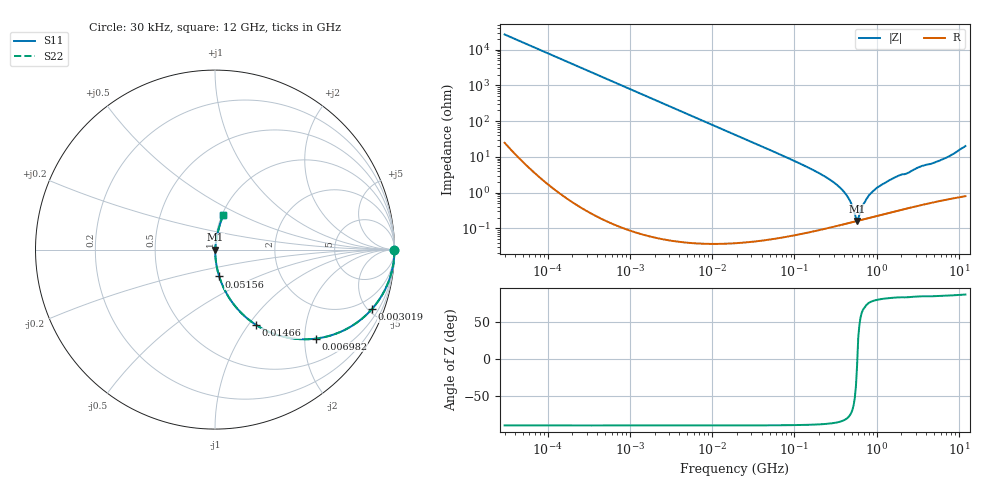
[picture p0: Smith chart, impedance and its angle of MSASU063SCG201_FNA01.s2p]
! MSASU063SCG201_FNA01  S-PARAMETER MODEL  ( General Type )
! Model Generated by TAIYO YUDEN Corporation (http://www.ty-top.com)
! Version 1.0
! TAIYO YUDEN Control No. 140905
! Copyright(c) 2014 TAIYO YUDEN CO.,LTD. All Rights Reserved.
! Product Description (link to TY-COMPAS)
! https://ds.yuden.co.jp/TYCOMPAS/or/detail?pn=MSASU063SCG201JFNA01&u=M
! Products Name : Multilayer Ceramic Capacitors
! Characteristics :
!  Capacitance : 200 pF , Rated Voltage : 50V , TCC : CG / C0G
!  Case Size : 0.6 x 0.3 / 0.024 x 0.012 [mm/inch] , Thickness : 0.3 / 0.012 [mm/inch]
!  (Conditions: Temperature = 25 degC , DC Bias Current/Voltage = 0A / 0V)
! External Node Assignments :
!  1  o---| |---o  2
! GND o---------o GND
! Frequency Range : 0.03MHz  -  12000MHz  [ 401 STEP ]
# MHz S RI R 50
! Freq[MHz].  S11 Real  S11 Imag  S21 Real  S21 Imag  S12 Real  S12 Imag  S22 Real  S22 Imag
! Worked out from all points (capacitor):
!   401 points, 30 kHz to 12 GHz, reference 50 ohm
!   read as one part in series: C = 200 pF near 32 kHz
!   lowest |Z| = 163 mohm at 579 MHz (marker M1)
!   series resonance near 582.7 MHz, so ESL is about 370 pH
!   S11 on the Smith chart (normalised r, x): 30 kHz: open; 3.019 MHz: 1.00, -5.26; 6.982 MHz: 1.00, -2.28; 14.66 MHz: 1.00, -1.08; 51.56 MHz: 1.00, -0.31; 12 GHz: 1.02, +0.40
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0.03  1 -0.00378  1.78e-05 0.00378  1.78e-05 0.00378  1 -0.00378
0.260295  0.9989 -0.0327  0.00108 0.0327  0.00108 0.0327  0.9989 -0.0327
0.886466  0.9877 -0.1102  0.0123 0.1102  0.0123 0.1102  0.9877 -0.1102
2.258455  0.9252 -0.263  0.0748 0.263  0.0748 0.263  0.9252 -0.263
3.018962  0.8738 -0.332  0.1262 0.332  0.1262 0.332  0.8738 -0.332
6.982189  0.5641 -0.4957  0.4359 0.4957  0.4359 0.4957  0.5641 -0.4957
14.65919  0.227 -0.4185  0.773 0.4185  0.773 0.4185  0.227 -0.4185
18.97367  0.1491 -0.3558  0.8509 0.3558  0.8509 0.3558  0.1491 -0.3558
51.55976  0.0233 -0.1493  0.9767 0.1493  0.9767 0.1493  0.0233 -0.1493
164.6252  0.00278 -0.0443  0.9972 0.0443  0.9972 0.0443  0.00278 -0.0443
275.7901  0.00156 -0.0223  0.9984 0.0223  0.9984 0.0223  0.00156 -0.0223
380.7415  0.00142 -0.012  0.9986 0.012  0.9986 0.012  0.00142 -0.012
462.0203  0.00146 -0.00645  0.9985 0.00645  0.9985 0.00645  0.00146 -0.00645
542.8588  0.00156 -0.00203  0.9984 0.00203  0.9984 0.00203  0.00156 -0.00203
579.0248  0.00161 -0.000227  0.9984 0.000227  0.9984 0.000227  0.00161 -0.000227
617.6002  0.00168 0.00176  0.9983 -0.00176  0.9983 -0.00176  0.00168 0.00176
725.66  0.00187 0.00536  0.9981 -0.00536  0.9981 -0.00536  0.00187 0.00536
852.6267  0.00211 0.00944  0.9979 -0.00944  0.9979 -0.00944  0.00211 0.00944
1428.372  0.00321 0.022  0.9968 -0.022  0.9968 -0.022  0.00321 0.022
3411.775  0.00725 0.053  0.9928 -0.053  0.9928 -0.053  0.00725 0.053
6715.658  0.0142 0.0887  0.9858 -0.0887  0.9858 -0.0887  0.0142 0.0887
12000  0.0459 0.1903  0.9541 -0.1903  0.9541 -0.1903  0.0459 0.1903
